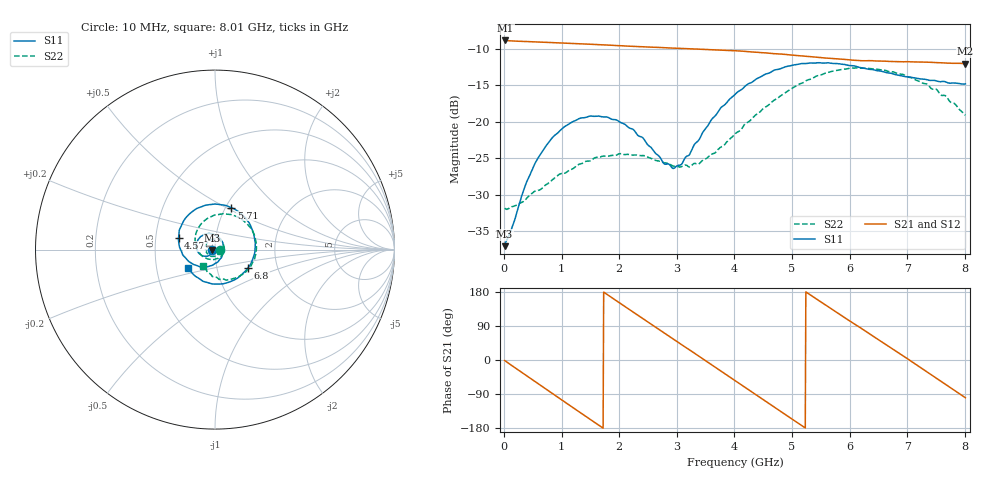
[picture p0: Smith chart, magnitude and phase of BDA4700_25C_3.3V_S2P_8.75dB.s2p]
!Agilent Technologies,E5071B,MY42404982,A.09.10
!Date: Mon Oct 20 18:06:40 2025
!Data & Calibration Information:
!Freq	S11:SOLT2(ON)	S21:SOLT2(ON)	S12:SOLT2(ON)	S22:SOLT2(ON)
# Hz S RI R 50
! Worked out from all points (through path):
!   801 points, 10 MHz to 8.01 GHz, reference 50 ohm
!   highest |S21| = -8.87 dB at 20 MHz (marker M1); lowest = -12.0 dB at 8.01 GHz (marker M2)
!   group delay of S21, straight-line fit = 283 ps
!   lowest |S11| = -37.0 dB at 10 MHz (marker M3), VSWR 1.03, Z = 48.6 - j0.151 ohm
!   |S11| at or under -10 dB: start of sweep to end of sweep
!   |S22| runs from -32.0 to -12.6 dB; largest |S21 - S12| = 0.0041
!   S11 on the Smith chart (normalised r, x): 10 MHz: 0.97, -0.00; 4.57 GHz: 0.66, +0.09; 5.71 GHz: 1.06, +0.53; 6.8 GHz: 1.41, -0.30; 8.01 GHz: 0.73, -0.16
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1e7  -0.014 -0.00155  0.3601 -0.00795  0.3601 -0.0081  0.0256 -0.0013
2e7  -0.0146 -0.00235  0.36 -0.0141  0.3597 -0.0149  0.0254 -0.00134
3.9e8  -0.0263 -0.0282  0.2654 -0.2345  0.2654 -0.2342  0.0201 -0.022
7.2e8  -0.0562 -0.0373  0.0845 -0.3394  0.0848 -0.3394  2.78e-05 -0.0369
1.02e9  -0.0878 -0.0224  -0.1025 -0.3304  -0.1024 -0.3304  -0.0274 -0.0347
1.35e9  -0.105 0.0163  -0.2672 -0.2124  -0.2674 -0.2126  -0.0512 -0.00716
1.93e9  -0.0593 0.0847  -0.3097 0.122  -0.3098 0.122  -0.0256 0.0529
2.32e9  0.000507 0.0809  -0.1562 0.2875  -0.1562 0.2875  0.0214 0.0551
2.68e9  0.0423 0.0406  0.0467 0.3193  0.046 0.3192  0.05 0.0202
2.96e9  0.0474 -0.00915  0.1912 0.2554  0.191 0.2549  0.0476 -0.0139
3.37e9  0.00734 -0.0737  0.3079 0.0616  0.3085 0.0617  0.0114 -0.0499
3.67e9  -0.0547 -0.0957  0.2929 -0.103  0.2929 -0.1038  -0.0299 -0.0539
4.01e9  -0.135 -0.0733  0.1783 -0.2489  0.1789 -0.2482  -0.076 -0.0316
4.57e9  -0.2033 0.0648  -0.1106 -0.274  -0.1099 -0.2745  -0.1099 0.066
4.98e9  -0.153 0.1879  -0.2568 -0.1262  -0.2573 -0.1274  -0.0676 0.1531
5.35e9  -0.04 0.2492  -0.2728 0.0558  -0.2731 0.0541  0.0239 0.1961
5.71e9  0.0901 0.2338  -0.1824 0.2002  -0.1821 0.2003  0.13 0.1801
6.18e9  0.2067 0.1121  0.0196 0.2613  0.0224 0.262  0.2226 0.0677
6.68e9  0.2059 -0.0643  0.2101 0.1509  0.2108 0.1507  0.2064 -0.0783
6.8e9  0.1842 -0.1007  0.2362 0.1041  0.2371 0.1025  0.1887 -0.1061
7.32e9  0.0371 -0.1914  0.224 -0.1236  0.2241 -0.1241  0.0663 -0.1695
8.01e9  -0.1491 -0.1037  -0.0417 -0.2468  -0.0409 -0.2471  -0.0649 -0.0896
